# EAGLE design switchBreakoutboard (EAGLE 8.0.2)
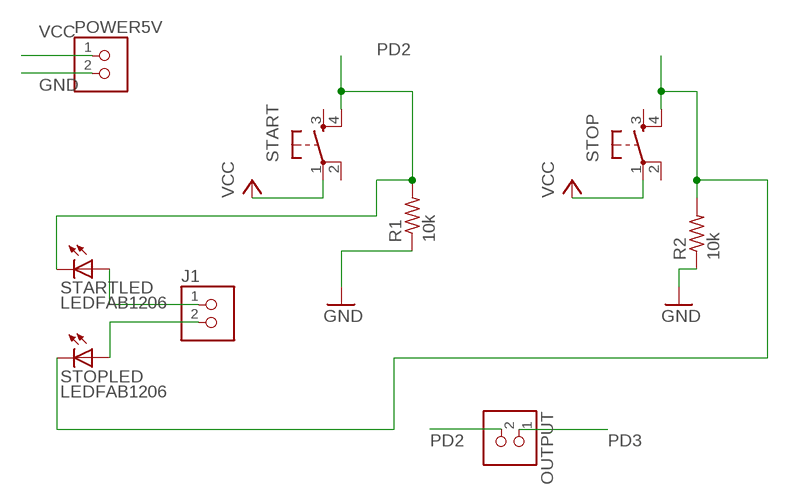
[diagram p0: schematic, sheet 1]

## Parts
J1  TERM-1X02-FABLAB  [ED555DS-2DS]
OUTPUT  TERM-1X02-ADAFRUIT  [3.5MMTERM]
POWER5V  TERM-1X02-FABLAB  [ED555DS-2DS]
R1  10k  RES-US1206FAB  [R1206FAB]
R2  10k  RES-US1206FAB  [R1206FAB]
START  6MM_SWITCH6MM_SWITCH  [6MM_SWITCH]
STARTLED  LEDFAB1206  [LED1206FAB]
STOP  6MM_SWITCH6MM_SWITCH  [6MM_SWITCH]
STOPLED  LEDFAB1206  [LED1206FAB]

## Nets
GND: POWER5V.2 R1.1 R2.1
PD2: OUTPUT.2 R1.2 START.4(S1) STARTLED.2(C)
PD3: OUTPUT.1 R2.2 STOP.4(S1) STOPLED.2(C)
PD6: J1.1 STARTLED.1(A)
PD7: J1.2 STOPLED.1(A)
VCC: POWER5V.1 START.1(P) STOP.1(P)
Unconnected: START.2(P1) START.3(S) STOP.2(P1) STOP.3(S)

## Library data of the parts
J1 OUTPUT POWER5V = fab:TERM-1X02: 3.5mm terminal block, 2 positions ED555-2DS as found in the fablab inventory.
R1 R2 = fab:RES-US: Resistor (US Symbol)
START STOP = fab:6MM_SWITCH: OMRON SWITCH
STARTLED STOPLED = fab:LED: LED

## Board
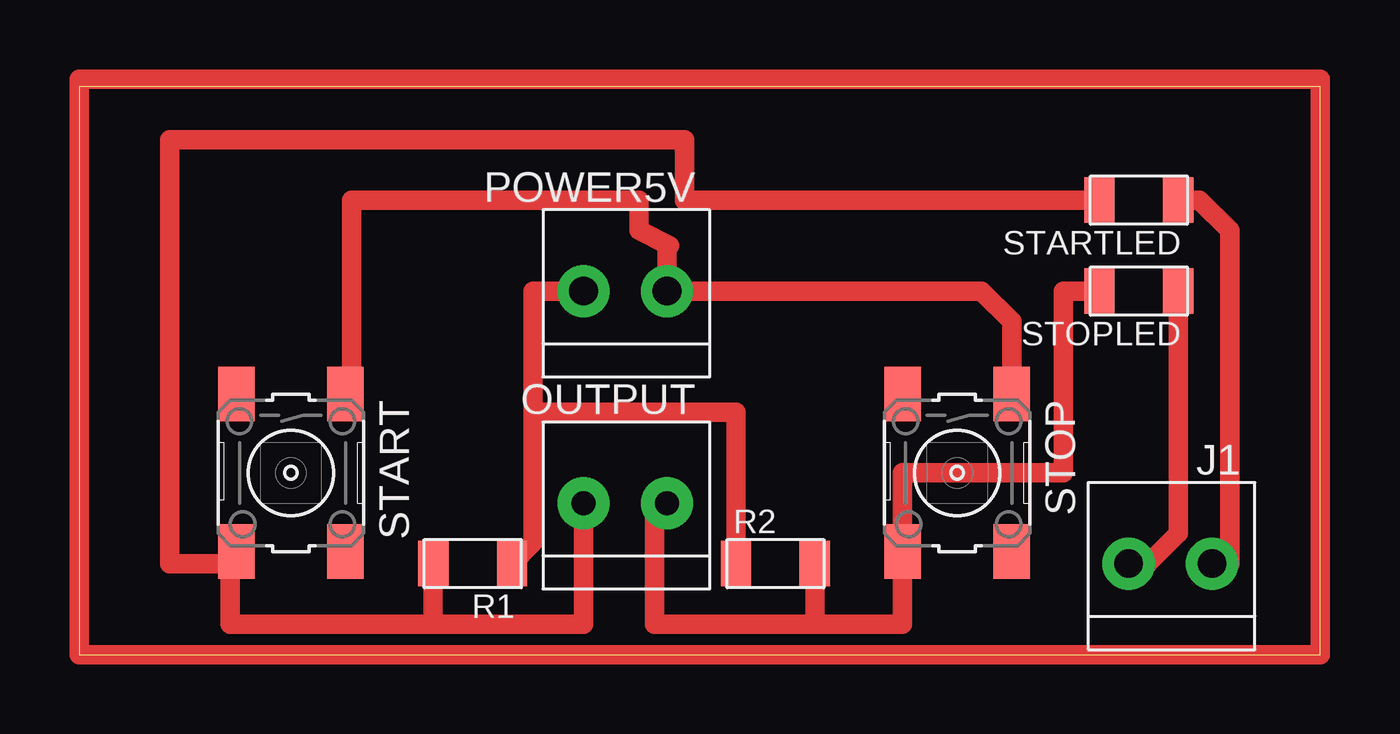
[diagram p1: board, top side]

Size 52.05 x 23.8 mm. Coordinates in mm from the lower left corner, seen from the top.
Outline: 0,0 52.05,0 52.05,23.8 0,23.8 0,0
Copper layers (1*16): Top 0.035mm / dielectric 1.5mm / Bottom 0.035mm
Design rules "default": minimum track width 10mil, minimum drill 24mil, track to track 8mil, track to pad 8mil, pad to pad 8mil, via to via 8mil, smd to smd 8mil, copper to edge 40mil, drill to drill 8mil, minimum pad ring 10mil, minimum via ring 8mil, stop-mask expansion 4mil, vias tented up to drill 0mil, thermal gap 10mil

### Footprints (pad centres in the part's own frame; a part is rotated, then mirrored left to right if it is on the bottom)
ED555DS-2DS = drill 1.2 pad 2.184: 1 1.8,0; 2 -1.7,0
3.5MMTERM = drill 1 pad 2.184: 1 1.8,0; 2 -1.7,0
R1206FAB = smd 1.27 x 1.905: 1 -1.651,0; 2 1.651,0
6MM_SWITCH = smd 2.286 x 1.524: 1 -3.302,2.286; 2 3.302,2.286; 3 -3.302,-2.286; 4 3.302,-2.286
LED1206FAB = smd 1.27 x 1.905: 1 -1.651,0; 2 1.651,0

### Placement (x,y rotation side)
J1  45.72,3.81 0 top
OUTPUT  22.86,6.35 0 top
POWER5V  22.86,15.24 0 top
R1  16.51,3.81 180 top
R2  29.21,3.81 0 top
START  8.89,7.62 270 top
STARTLED  44.45,19.05 180 top
STOP  36.83,7.62 270 top
STOPLED  44.45,15.24 180 top

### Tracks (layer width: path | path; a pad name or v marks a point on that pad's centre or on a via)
GND
  Top 0.254: 18.19,4 R1.1
  Top 0.813: R1.1 19.05,4.7 19.05,10.16 | 19.05,10.16 19.05,15.24 POWER5V.2 | 19.05,10.16 27.56,10.16 R2.1
N$1
  Top 0.813: 0,0 52.07,0 52.07,24.13 0,24.13 0,0
PD2
  Top 0.254: R1.2 14.71,3.89
  Top 0.813: STARTLED.2 25.4,19.05 25.4,21.59 3.81,21.59 3.81,3.81 6.6,3.81 START.4 6.35,4.32 6.35,1.27 14.86,1.27 | 14.86,1.27 R1.2 | 14.86,1.27 21.16,1.27 OUTPUT.2
PD3
  Top 0.813: OUTPUT.1 24.13,6.35 24.13,1.27 30.86,1.27 | 30.86,1.27 R2.2 | 30.86,1.27 34.54,1.27 STOP.4 34.54,7.62 41.27,7.62 41.27,15.24 STOPLED.2
PD6
  Top 0.813: STARTLED.1 46.99,19.05 48.26,17.78 48.26,3.81 J1.1
PD7
  Top 0.813: J1.2 44.83,3.81 46.1,5.08 STOPLED.1
VCC
  Top 0.813: STOP.1 39.12,13.97 37.85,15.24 POWER5V.1 24.66,17.04 24.77,17.14 23.5,17.78 23.5,19.05 11.43,19.05 11.43,11.18 START.1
